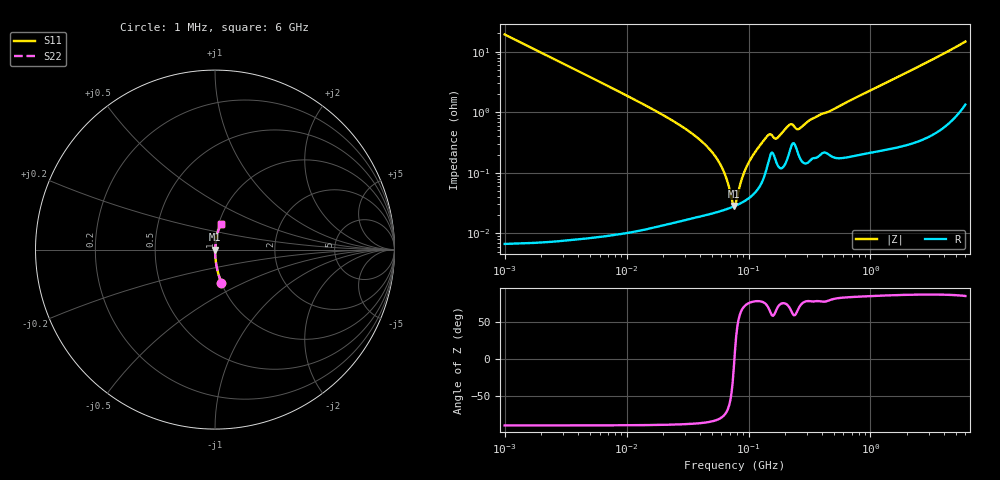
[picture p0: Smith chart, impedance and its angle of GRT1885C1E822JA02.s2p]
!Murata Part Number: GRT1885C1E822JA02
!These Parameters are Measured in Series Mode Connection
!Data Generated on Jun 19, 2026
!  o--ll--o
!Port1  Port2
!  o------o
!Operation Temp=25[degC], DC Bias Voltage=0[V]
!Freq. Start=1000[kHz] Stop=6[GHz] 401[Steps]
# Hz S RI R 50
!Freq.(Hz) S11(Real) S11(Imag) S21(Real) S21(Imag) S12(Real) S12(Imag) S22(Real) S22(Imag)
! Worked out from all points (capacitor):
!   401 points, 1 MHz to 6 GHz, reference 50 ohm
!   read as one part in series: C = 8.26 nF near 1.044 MHz
!   lowest |Z| = 28.4 mohm at 75.79 MHz (marker M1)
!   series resonance near 76.62 MHz, so ESL is about 520 pH
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1000000  0.0359 -0.1858  0.9641 0.1858  0.9641 0.1858  0.0359 -0.1858
4293785  0.00208 -0.0446  0.9979 0.0446  0.9979 0.0446  0.00208 -0.0446
1.843659e7  0.000226 -0.00981  0.9998 0.00981  0.9998 0.00981  0.000226 -0.00981
3.389622e7  0.000195 -0.00455  0.9998 0.00455  0.9998 0.00455  0.000195 -0.00455
5.013812e7  0.000217 -0.0022  0.9998 0.0022  0.9998 0.0022  0.000217 -0.0022
6.23192e7  0.000242 -0.00105  0.9998 0.00105  0.9998 0.00105  0.000242 -0.00105
6.652088e7  0.000253 -0.000718  0.9997 0.000718  0.9997 0.000718  0.000253 -0.000718
7.256705e7  0.000269 -0.000276  0.9997 0.000276  0.9997 0.000276  0.000269 -0.000276
7.57932e7  0.000279 -5.51e-05  0.9997 5.51e-05  0.9997 5.51e-05  0.000279 -5.51e-05
7.745967e7  0.000284 5.58e-05  0.9997 -5.58e-05  0.9997 -5.58e-05  0.000284 5.58e-05
7.916277e7  0.000289 0.000167  0.9997 -0.000167  0.9997 -0.000167  0.000289 0.000167
9.019724e7  0.000331 0.000847  0.9997 -0.000847  0.9997 -0.000847  0.000331 0.000847
9.83954e7  0.00037 0.00132  0.9996 -0.00132  0.9996 -0.00132  0.00037 0.00132
1.121107e8  0.000465 0.00209  0.9995 -0.00209  0.9995 -0.00209  0.000465 0.00209
1.39348e8  0.0011 0.00367  0.9989 -0.00367  0.9989 -0.00367  0.0011 0.00367
1.487431e8  0.00181 0.00393  0.9982 -0.00393  0.9982 -0.00393  0.00181 0.00393
1.694764e8  0.00148 0.00337  0.9985 -0.00337  0.9985 -0.00337  0.00148 0.00337
2.152823e8  0.00214 0.00575  0.9979 -0.00575  0.9979 -0.00575  0.00214 0.00575
2.561955e8  0.00204 0.00484  0.998 -0.00484  0.998 -0.00484  0.00204 0.00484
3.325952e8  0.00177 0.00759  0.9982 -0.00759  0.9982 -0.00759  0.00177 0.00759
1.428092e9  0.0035 0.0324  0.9965 -0.0324  0.9965 -0.0324  0.0035 0.0324
6e9  0.0335 0.1399  0.9665 -0.1399  0.9665 -0.1399  0.0335 0.1399
